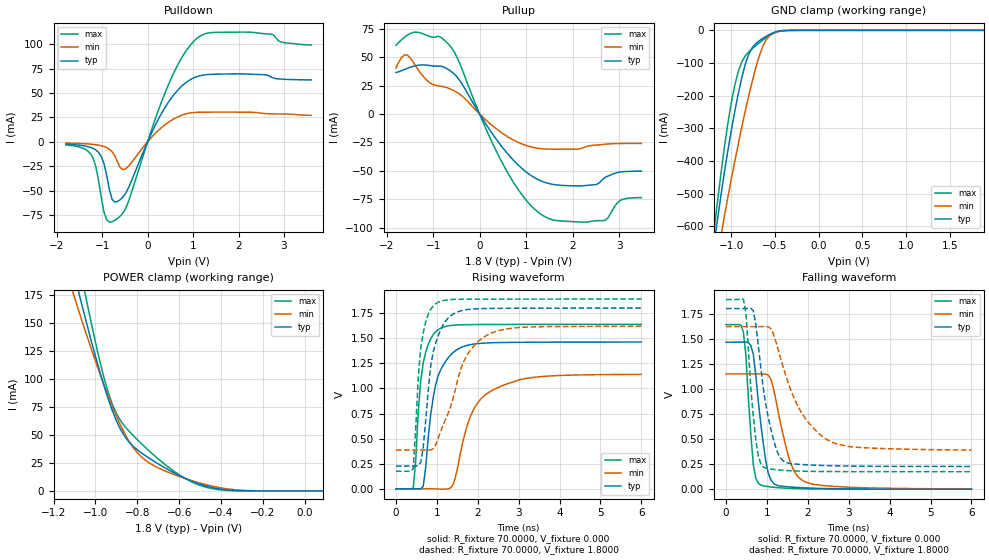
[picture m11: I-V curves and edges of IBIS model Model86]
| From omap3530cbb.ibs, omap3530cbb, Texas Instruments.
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| Model based on original model for BQ0247S_7LM
|   Sub model BQ0247S_7LM_18PD
[model]   Model86
|[Input Load]   PD
|[Output Drive]
|Voltage   1.8000V
|Mode   I/O
Model_type   I/O
Polarity   Non-Inverting
Enable   Active-Low
Vinl =   0.6615V
Vinh =   1.0530V
Vmeas =   0.9000V
Cref =  15.0000pF
Rref =  70.0000
Vref =  0.000V
C_comp   14.0442pF   14.1784pF   14.5599pF
[Temperature Range]   25.0000   0.1250k   -40.0000
[Voltage Range]   1.8000V   1.6200V   1.8900V
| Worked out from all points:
|   slope of the pulldown table from 0 to 0.27 V, typ, clamps not added: 10.4 ohm
|   slope of the pullup table from 0 to 0.27 V, typ, clamps not added: 15.9 ohm
|   GND clamp passes 1 mA (typ) near -0.41 V on its own axis
|   POWER clamp passes 1 mA (typ) near -0.37 V on its own axis
|   rising waveform, R_fixture 70.0000, V_fixture 0.000: 20-80 % time 334ps typ, 601ps min, 210ps max; typ from 0 V to 1.46 V
|   rising waveform, R_fixture 70.0000, V_fixture 1.8000: 20-80 % time 304ps typ, 655ps min, 193ps max; typ from 0.226 V to 1.8 V
|   falling waveform, R_fixture 70.0000, V_fixture 0.000: 20-80 % time 250ps typ, 405ps min, 162ps max; typ from 1.47 V to 0.001 V
|   falling waveform, R_fixture 70.0000, V_fixture 1.8000: 20-80 % time 356ps typ, 788ps min, 201ps max; typ from 1.8 V to 0.227 V
[Pulldown]
-1.8V     -2.315mA   -1.247mA   -3.18mA
-1.26V    -5.735mA   -2.395mA   -12.01mA
-1.14V    -8.407mA   -3.014mA   -25.29mA
-1.02V    -15.01mA   -4.055mA   -57.13mA
-900mV    -34.53mA   -5.974mA   -79.95mA
-780mV    -59.24mA   -10.29mA   -82.04mA
-480mV    -52.65mA   -27.56mA   -68.16mA
420mV     37.97mA    18.77mA    54.35mA
780mV     58.41mA    27.78mA    88.55mA
1.08V     66.8mA     30.24mA    106mA
2.28V     69.36mA    30.28mA    112.4mA
3.6V      63.53mA    27.1mA     99.3mA
[Pullup]
-1.8V     36.49mA    40.41mA    60.33mA
-1.56V    40.02mA    51.79mA    69.09mA
-1.08V    42.61mA    27.69mA    68.26mA
-660mV    38.74mA    22.49mA    60.94mA
-480mV    32.28mA    18.83mA    49.4mA
540mV     -31.82mA   -18.28mA   -46.84mA
960mV     -49.54mA   -27.06mA   -73.55mA
1.38V     -59.71mA   -30.65mA   -89.61mA
2.22V     -63.07mA   -29.86mA   -94.98mA
2.7V      -55.69mA   -26.56mA   -93.38mA
3V        -51.12mA   -25.94mA   -76.6mA
3.48V     -50.1mA    -25.83mA   -73.43mA
[GND_clamp]
-1.8V     -1.9A      -1.807A    -2.065A
-1.2V     -659.6mA   -761.2mA   -618.3mA
-1.16V    -582.8mA   -696.2mA   -528.9mA
-1.12V    -508.3mA   -632.8mA   -442.5mA
-1.08V    -436.9mA   -571.4mA   -360.9mA
-1V       -307.1mA   -455.6mA   -221.8mA
-920mV    -194.8mA   -348.2mA   -126.3mA
-800mV    -73.12mA   -200.3mA   -66.1mA
-680mV    -32.03mA   -78.98mA   -38.42mA
-600mV    -18.23mA   -28.9mA    -21.92mA
-360mV    -301.2uA   -671.4uA   -205.9uA
1.89V     0A         0A         0A
[POWER_clamp]
-1.8V     791.2mA    693.9mA    1.001A
-1.1V     193mA      173.2mA    224.6mA
-1.08V    177.9mA    161.4mA    205.4mA
-1.06V    163.1mA    149.8mA    186.6mA
-1.04V    148.6mA    138.4mA    168.2mA
-960mV    94.77mA    95.29mA    102.1mA
-900mV    62.97mA    66.99mA    69.41mA
-800mV    36.81mA    34.25mA    45.87mA
-680mV    22mA       18.94mA    25.57mA
-560mV    10.38mA    10.44mA    9.994mA
-440mV    2.953mA    4.194mA    1.993mA
90mV      0A         0A         0A
[Ramp]
dV/dt_r   0.8770/0.3308n   0.6836/0.5954n   0.9830/0.2079n
dV/dt_f   0.9436/0.3524n   0.7372/0.7798n   1.0290/0.1986n
R_load = 70.0000
[Rising Waveform]
R_fixture = 70.0000
V_fixture = 0.000
V_fixture_min = 0.000
V_fixture_max = 0.000
0s        306.8uV    369.2uV    306.5uV
424.2ps   236uV      359uV      7.589mV
545.5ps   -297.8uV   362.8uV    764.8mV
666.7ps   22.93mV    304.4uV    1.254V
848.5ps   732.9mV    46.73uV    1.494V
1.03ns    1.124V     -2.233mV   1.585V
1.394ns   1.355V     40.45mV    1.629V
1.818ns   1.436V     718.3mV    1.635V
2.303ns   1.454V     968.3mV    1.637V
6ns       1.462V     1.14V      1.639V
[Rising Waveform]
R_fixture = 70.0000
V_fixture = 1.8000
V_fixture_min = 1.6200
V_fixture_max = 1.8900
0s        226.5mV    386.2mV    174.6mV
424.2ps   226.6mV    386.3mV    200mV
545.5ps   229mV      386.4mV    1.101V
606.1ps   264.7mV    386.4mV    1.4V
848.5ps   1.221V     387.7mV    1.786V
969.7ps   1.447V     437.3mV    1.842V
1.212ns   1.669V     691.2mV    1.879V
1.636ns   1.778V     1.249V     1.888V
2.182ns   1.796V     1.519V     1.889V
6ns       1.8V       1.619V     1.89V
[Falling Waveform]
R_fixture = 70.0000
V_fixture = 0.000
V_fixture_min = 0.000
V_fixture_max = 0.000
0s        1.465V     1.149V     1.64V
424.2ps   1.465V     1.149V     1.565V
484.8ps   1.465V     1.149V     1.333V
666.7ps   1.343V     1.149V     246.9mV
848.5ps   654.4mV    1.149V     41.64mV
969.7ps   284.9mV    1.146V     29.41mV
1.091ns   97.09mV    1.101V     22.66mV
1.576ns   21.99mV    264.2mV    8.19mV
1.879ns   14.61mV    85.37mV    4.443mV
6ns       893.8uV    3.168mV    602.6uV
[Falling Waveform]
R_fixture = 70.0000
V_fixture = 1.8000
V_fixture_min = 1.6200
V_fixture_max = 1.8900
0s        1.8V       1.62V      1.89V
424.2ps   1.8V       1.62V      1.895V
484.8ps   1.8V       1.62V      1.758V
666.7ps   1.778V     1.62V      723.9mV
787.9ps   1.438V     1.62V      332mV
909.1ps   1.01V      1.62V      223.3mV
1.333ns   310.1mV    1.304V     190.3mV
1.818ns   247.1mV    780.5mV    180.1mV
2.485ns   234.9mV    490mV      176.3mV
6ns       227.2mV    391.1mV    174.9mV
